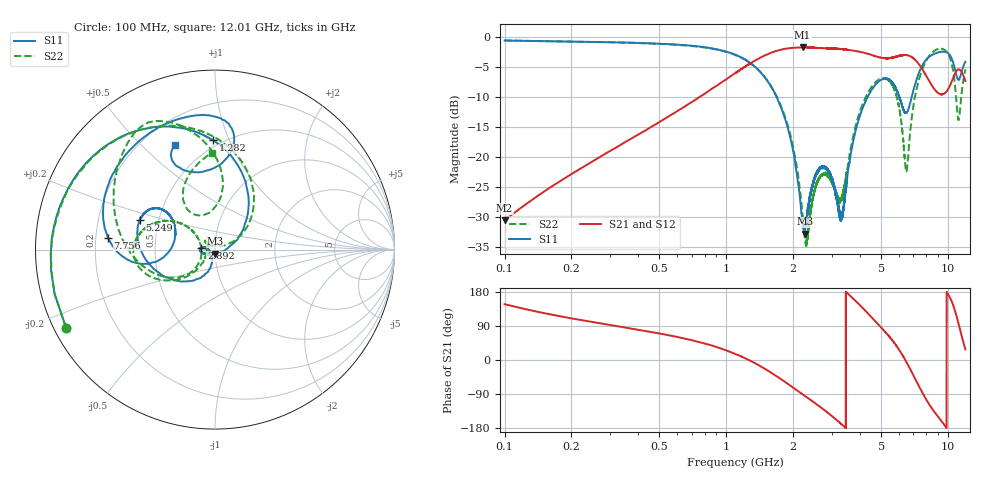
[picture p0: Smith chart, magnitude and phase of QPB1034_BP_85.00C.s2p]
! TDS: k:\Engsetup\Winsaw\QPB1034_ALL
! Channel 1
! Ports=1 2
! seg 1=100.000000 1100.000000 51
! seg 2=1101.000000 1301.000000 201
! seg 3=1302.000000 2302.000000 101
! seg 4=2303.000000 3503.000000 1201
! seg 5=3504.000000 5204.000000 171
! seg 6=5205.000000 6405.000000 1201
! seg 7=6406.000000 8506.000000 211
! seg 8=8507.000000 12007.000000 176
! Points=3313
! FailCode=0
! Topology=ALL_SE(12)
!VNA Cal loaded =QPB1034_ALL_85C
!PS1(V)= 5.000
!PS(mA)= 0.601
!PS2(V)= 1.170
!PS(mA)= -0.001
!PS3(V)= 1.170
!PS(mA)= 0.000
!PS4(V)= 1.170
!PS(mA)= -0.001
!Temp (C)= 85.00
# MHz S DB R 50
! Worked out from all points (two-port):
!   3313 points, 100 MHz to 12.01 GHz, reference 50 ohm
!   highest |S21| = -1.71 dB at 2.212 GHz (marker M1); lowest = -30.6 dB at 100 MHz (marker M2)
!   |S21| within 3 dB of the highest: 1.243 GHz to 7.474 GHz (6.231 GHz wide, 143 % of centre)
!   lowest |S11| = -32.8 dB at 2.262 GHz (marker M3), VSWR 1.05, Z = 50 - j2.29 ohm
!   |S11| at or under -10 dB: 1.689 GHz to 4.341 GHz (2.652 GHz wide, 88 % of centre); 6.043 GHz to 6.871 GHz (827.1 MHz wide, 12.8 % of centre)
!   |S22| runs from -34.9 to -0.6 dB; largest |S21 - S12| = 0.0068
!   S11 on the Smith chart (normalised r, x): 100 MHz: 0.03, -0.25; 1.282 GHz: 0.45, +0.87; 2.892 GHz: 0.86, +0.02; 5.249 GHz: 0.39, +0.16; 7.756 GHz: 0.25, +0.05; 12.01 GHz: 0.33, +0.63
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100  -0.57 -152.3  -30.55 147.2  -30.54 147.0  -0.56 -152.3
240  -0.79 178.6  -21.11 101.8  -21.11 101.7  -0.81 179.0
500  -1.10 154.5  -14.17 70.0  -14.17 70.0  -1.12 154.9
1100  -2.95 107.2  -5.97 16.1  -5.99 16.0  -2.98 104.7
1282  -4.30 91.0  -4.41 -1.7  -4.42 -2.0  -4.32 87.4
1812  -12.86 41.6  -2.01 -54.8  -2.00 -54.8  -12.52 37.6
2212  -30.54 -47.7  -1.71 -90.3  -1.74 -90.2  -29.69 38.1
2262  -32.82 -89.3  -1.72 -94.3  -1.73 -94.4  -33.67 60.8
2434  -25.12 -152.8  -1.77 -107.6  -1.74 -107.7  -28.03 140.6
2892  -22.33 172.2  -1.88 -140.5  -1.88 -140.5  -23.20 138.3
3313  -30.44 -146.2  -2.00 -169.5  -1.99 -169.4  -27.20 -173.1
3994  -13.32 -126.6  -2.43 145.9  -2.44 145.8  -12.67 -138.0
5249  -6.95 158.7  -3.51 72.5  -3.52 72.4  -6.90 176.9
5406  -7.05 153.0  -3.52 63.9  -3.49 63.9  -7.22 170.7
5998  -9.70 142.5  -3.14 29.1  -3.17 29.2  -11.25 144.9
6456  -12.66 164.9  -3.01 -1.9  -2.98 -2.1  -22.00 168.1
7106  -7.97 -168.5  -3.76 -48.3  -3.75 -48.3  -9.98 -151.1
7756  -4.43 173.6  -5.63 -90.8  -5.63 -90.8  -4.96 165.3
9047  -2.56 119.2  -9.34 -149.9  -9.32 -150.0  -1.98 122.7
10447  -3.73 80.7  -7.27 152.7  -7.29 152.7  -4.62 94.5
11187  -7.15 99.5  -5.37 95.3  -5.36 95.6  -13.86 107.2
12007  -4.12 111.0  -7.34 28.0  -7.36 28.1  -5.38 91.8
